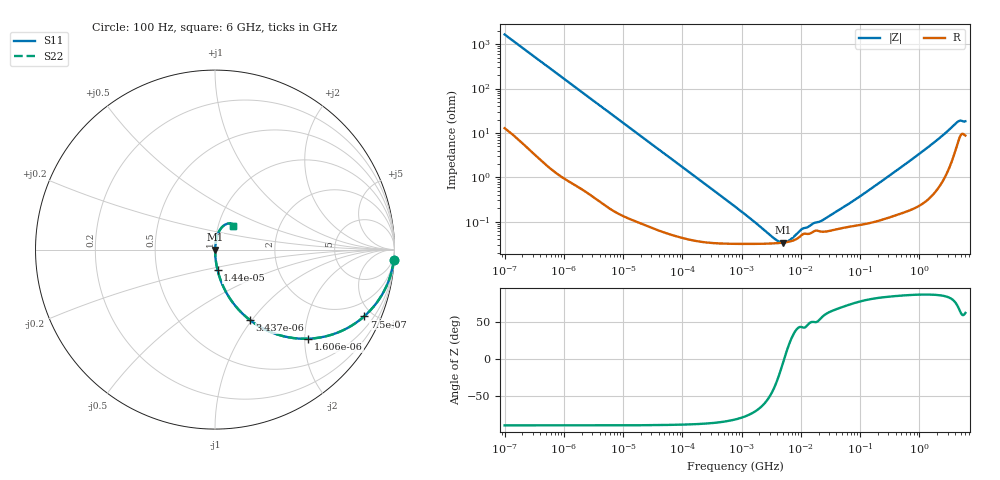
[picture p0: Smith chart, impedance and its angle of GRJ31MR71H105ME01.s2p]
!Murata Part Number: GRJ31MR71H105ME01
!These Parameters are Measured in Series Mode Connection
!Data Generated on Jun 19, 2026
!  o--ll--o
!Port1  Port2
!  o------o
!Operation Temp=25[degC], DC Bias Voltage=0[V]
!Freq. Start=100[Hz] Stop=6[GHz] 401[Steps]
# Hz S RI R 50
!Freq.(Hz) S11(Real) S11(Imag) S21(Real) S21(Imag) S12(Real) S12(Imag) S22(Real) S22(Imag)
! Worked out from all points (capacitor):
!   401 points, 100 Hz to 6 GHz, reference 50 ohm
!   read as one part in series: C = 959 nF near 109 Hz
!   lowest |Z| = 33.8 mohm at 5.079 MHz (marker M1)
!   series resonance near 5.256 MHz, so ESL is about 960 pH
!   S11 on the Smith chart (normalised r, x): 100 Hz: 1, -33; 750 Hz: 1.02, -4.45; 1.606 kHz: 1.01, -2.08; 3.437 kHz: 1.01, -0.98; 14.4 kHz: 1.00, -0.23; 6 GHz: 1.17, +0.32
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100  0.9959 -0.0601  0.0041 0.0601  0.0041 0.0601  0.9959 -0.0601
350  0.9565 -0.2009  0.0435 0.2009  0.0435 0.2009  0.9565 -0.2009
750  0.8307 -0.3723  0.1693 0.3723  0.1693 0.3723  0.8307 -0.3723
1606  0.5205 -0.4965  0.4795 0.4965  0.4795 0.4965  0.5205 -0.4965
2008  0.4108 -0.4888  0.5892 0.4888  0.5892 0.4888  0.4108 -0.4888
3437  0.1942 -0.3923  0.8058 0.3923  0.8058 0.3923  0.1942 -0.3923
6151  0.0711 -0.2535  0.9289 0.2535  0.9289 0.2535  0.0711 -0.2535
14402  0.0146 -0.1153  0.9854 0.1153  0.9854 0.1153  0.0146 -0.1153
40335  0.00239 -0.0419  0.9976 0.0419  0.9976 0.0419  0.00239 -0.0419
774597  0.00032 -0.00216  0.9997 0.00216  0.9997 0.00216  0.00032 -0.00216
3549919  0.000324 -0.000263  0.9997 0.000263  0.9997 0.000263  0.000324 -0.000263
5079039  0.000337 -2.24e-05  0.9997 2.24e-05  0.9997 2.24e-05  0.000337 -2.24e-05
6353432  0.000354 0.000126  0.9996 -0.000126  0.9996 -0.000126  0.000354 0.000126
1.039699e7  0.0005 0.000458  0.9995 -0.000458  0.9995 -0.000458  0.0005 0.000458
1.555665e7  0.000572 0.000668  0.9994 -0.000668  0.9994 -0.000668  0.000572 0.000668
2.327686e7  0.000592 0.000897  0.9994 -0.000897  0.9994 -0.000897  0.000592 0.000897
5.449875e7  0.000736 0.00206  0.9993 -0.00206  0.9993 -0.00206  0.000736 0.00206
3.124326e8  0.00136 0.0108  0.9986 -0.0108  0.9986 -0.0108  0.00136 0.0108
1.497423e9  0.00594 0.0504  0.9941 -0.0504  0.9941 -0.0504  0.00594 0.0504
4.193612e9  0.0658 0.1433  0.9342 -0.1433  0.9342 -0.1433  0.0658 0.1433
4.796499e9  0.096 0.1427  0.904 -0.1427  0.904 -0.1427  0.096 0.1427
6e9  0.0999 0.1333  0.9001 -0.1333  0.9001 -0.1333  0.0999 0.1333
